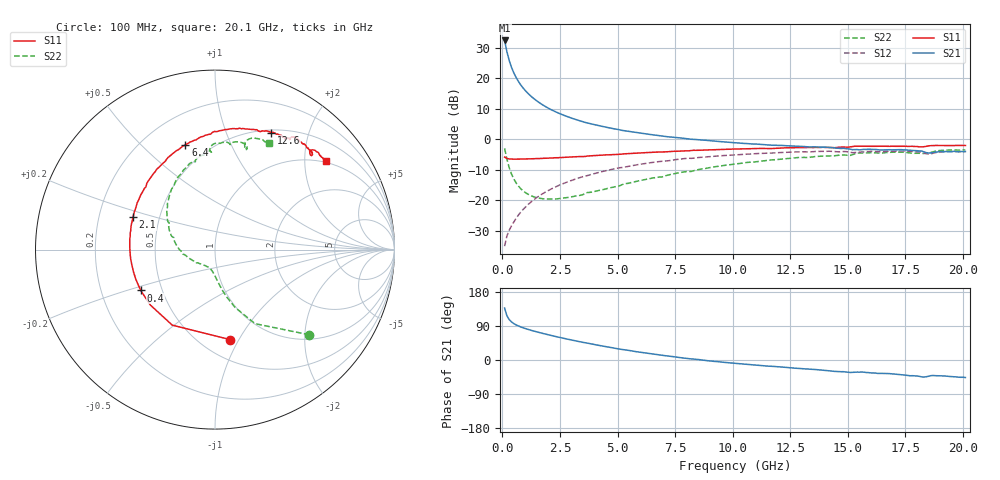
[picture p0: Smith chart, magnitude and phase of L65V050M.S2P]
!  Infineon Technologies AG
! BFR380L3 , PF131585-7, No.6, Th 09.10.01, soldered on pcb-board, measured with PP GSG850
!  Vce=5.0 V,  Ic=50.0 mA
! Common Emitter S-Parameters:  15. November 2001
#  GHz  S  MA  R  50
! f  S11  S21  S12  S22
! GHz  Mag  Ang  Mag  Ang  Mag  Ang  Mag  Ang
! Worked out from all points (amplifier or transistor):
!   201 points, 100 MHz to 20.1 GHz, reference 50 ohm
!   highest |S21| = 32.4 dB at 100 MHz (marker M1)
!   |S21| within 3 dB of that: start of sweep to 181 MHz
!   unconditionally stable (mu >= 1): 981.4 MHz to 4.293 GHz
!   at 3.4 GHz: K = 1.02, MAG = 8.4 dB, |S12| = -12.5 dB
!   at 10.1 GHz: K = 0.95, MSG = 2.0 dB, |S12| = -5.1 dB
!   at 20.1 GHz: K = 0.99, MSG = 0.0 dB, |S12| = -4.1 dB
!   S11 on the Smith chart (normalised r, x): 100 MHz: 0.68, -0.92; 400 MHz: 0.38, -0.22; 2.1 GHz: 0.35, +0.17; 6.4 GHz: 0.37, +0.69; 12.6 GHz: 0.53, +1.45; 20.1 GHz: 0.97, +2.53
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0.1  0.5085 -80.4  41.71 137.0  0.01759 63.3  0.7084 -42.1
0.2  0.4835 -119.5  27.23 116.6  0.0259 57.6  0.4693 -61.6
0.3  0.4745 -139.3  19.52 106.6  0.03209 58.8  0.341 -70.9
0.4  0.4724 -151.2  15.08 100.4  0.03805 61.1  0.2682 -76.5
0.5  0.4709 -159.1  12.23 96.0  0.04399 63.3  0.2228 -80.4
0.6  0.4709 -164.7  10.28 92.6  0.05054 64.9  0.1923 -83.5
0.7  0.471 -169.5  8.867 89.8  0.05694 66.0  0.1703 -86.2
0.9  0.4733 -176.7  6.946 85.0  0.0703 67.6  0.1423 -90.8
1.1  0.4752 177.9  5.723 81.1  0.08374 68.3  0.1263 -95.4
1.4  0.4784 171.0  4.533 75.8  0.104 68.2  0.1125 -101.8
1.7  0.4848 165.0  3.762 71.0  0.1243 67.4  0.1062 -108.4
2.1  0.4924 158.3  3.08 65.0  0.1513 65.9  0.1046 -116.8
2.7  0.5058 149.0  2.445 56.7  0.1911 62.7  0.1089 -129.9
3.5  0.5197 137.9  1.936 46.5  0.2433 57.7  0.1234 -143.4
4.9  0.5617 121.2  1.469 30.8  0.3284 48.5  0.1658 -168.6
6.4  0.6053 105.8  1.199 16.7  0.4103 38.2  0.2264 169.8
6.8  0.6161 102.1  1.144 13.3  0.4298 35.2  0.2393 164.5
10.1  0.6893 77.7  0.8741 -8.8  0.555 13.4  0.3919 130.5
12.6  0.7233 64.4  0.773 -20.8  0.6149 -2.3  0.4896 108.3
13.5  0.7304 60.3  0.7498 -24.7  0.6252 -7.7  0.5137 101.8
16.8  0.7638 47.9  0.6724 -35.9  0.6336 -24.0  0.6087 79.8
20.1  0.7889 38.6  0.6284 -46.2  0.6272 -38.0  0.6687 63.0
